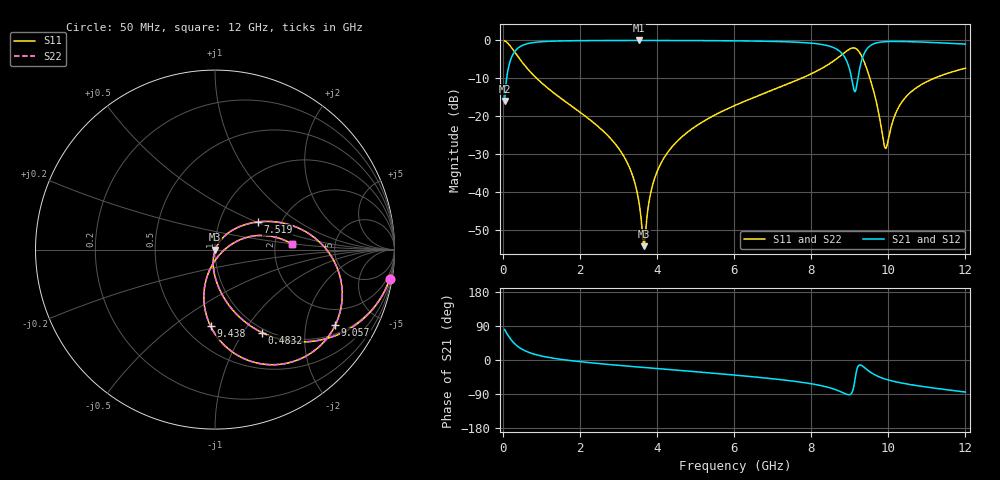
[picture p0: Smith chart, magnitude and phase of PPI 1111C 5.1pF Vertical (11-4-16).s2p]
# GHz S MA R 50
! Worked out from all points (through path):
!   1601 points, 50 MHz to 12 GHz, reference 50 ohm
!   highest |S21| = -0.02 dB at 3.53 GHz (marker M1); lowest = -15.9 dB at 50 MHz (marker M2)
!   group delay of S21, straight-line fit = 23.5 ps
!   lowest |S11| = -54.2 dB at 3.665 GHz (marker M3), VSWR 1.00, Z = 50.2 - j0.0591 ohm
!   |S11| at or under -10 dB: 881.8 MHz to 7.745 GHz (6.863 GHz wide, 159 % of centre); 9.524 GHz to 11.19 GHz (1.662 GHz wide, 16.1 % of centre)
!   |S22| runs from -54.2 to -0.1 dB; largest |S21 - S12| = 0
!   S11 on the Smith chart (normalised r, x): 50 MHz: 1, -12; 483.2 MHz: 0.95, -1.22; 7.519 GHz: 1.52, +0.51; 9.057 GHz: 1.31, -2.94; 9.438 GHz: 0.66, -0.69; 12 GHz: 2.49, +0.19
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0.05  0.9871 -9.5  0.1598 80.5  0.1598 80.5  0.9871 -9.5
0.2143125  0.8208 -36.0  0.5709 54.0  0.5709 54.0  0.8208 -36.0
0.4831875  0.533 -60.4  0.8454 29.6  0.8454 29.6  0.533 -60.4
2.044156  0.1094 -94.1  0.9925 -4.8  0.9925 -4.8  0.1094 -94.1
3.082313  0.03322 -101.7  0.9975 -14.8  0.9975 -14.8  0.03322 -101.7
3.530438  0.007596 -94.2  0.9979 -18.6  0.9979 -18.6  0.007596 -94.2
3.664875  0.001945 -17.6  0.9978 -19.7  0.9978 -19.7  0.001945 -17.6
3.844125  0.01005 57.2  0.9977 -21.2  0.9977 -21.2  0.01005 57.2
4.038312  0.02046 61.3  0.9975 -22.9  0.9975 -22.9  0.02046 61.3
4.725437  0.05796 59.1  0.9957 -28.6  0.9957 -28.6  0.05796 59.1
6.025  0.1392 48.8  0.9867 -39.9  0.9867 -39.9  0.1392 48.8
7.51875  0.2827 33.0  0.9518 -55.6  0.9518 -55.6  0.2827 33.0
8.019156  0.3662 25.1  0.9178 -63.0  0.9178 -63.0  0.3662 25.1
8.691344  0.5879 3.7  0.751 -80.5  0.751 -80.5  0.5879 3.7
9.057313  0.7912 -32.1  0.3029 -86.2  0.3029 -86.2  0.7912 -32.1
9.139469  0.7887 -45.9  0.2111 -49.6  0.2111 -49.6  0.7887 -45.9
9.236562  0.716 -63.6  0.3729 -14.2  0.3729 -14.2  0.716 -63.6
9.438219  0.4281 -93.3  0.761 -24.5  0.761 -24.5  0.4281 -93.3
9.893812  0.04189 -66.5  0.9594 -49.4  0.9594 -49.4  0.04189 -66.5
10.01331  0.05306 -0.4  0.9664 -53.0  0.9664 -53.0  0.05306 -0.4
10.566  0.2044 20.5  0.9617 -64.8  0.9617 -64.8  0.2044 20.5
12  0.4301 4.2  0.8926 -84.5  0.8926 -84.5  0.4301 4.2
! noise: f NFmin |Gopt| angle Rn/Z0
0.05  0.0004569  0.9017  2.419  0.001017
1.372  0.003956  0.6886  8.273  0.002458
2.701  0.006504  0.641  14.96  0.003368
4.031  0.008937  0.6212  21.53  0.004259
5.36  0.01167  0.6228  27.88  0.005464
6.682  0.01587  0.6569  34.1  0.008099
8.012  0.03002  0.7747  40.75  0.02398
9.341  0.1742  0.9519  47.68  0.6805
10.67  0.03679  0.7727  53.03  0.02656
12  0.0313  0.7216  57.56  0.01726
